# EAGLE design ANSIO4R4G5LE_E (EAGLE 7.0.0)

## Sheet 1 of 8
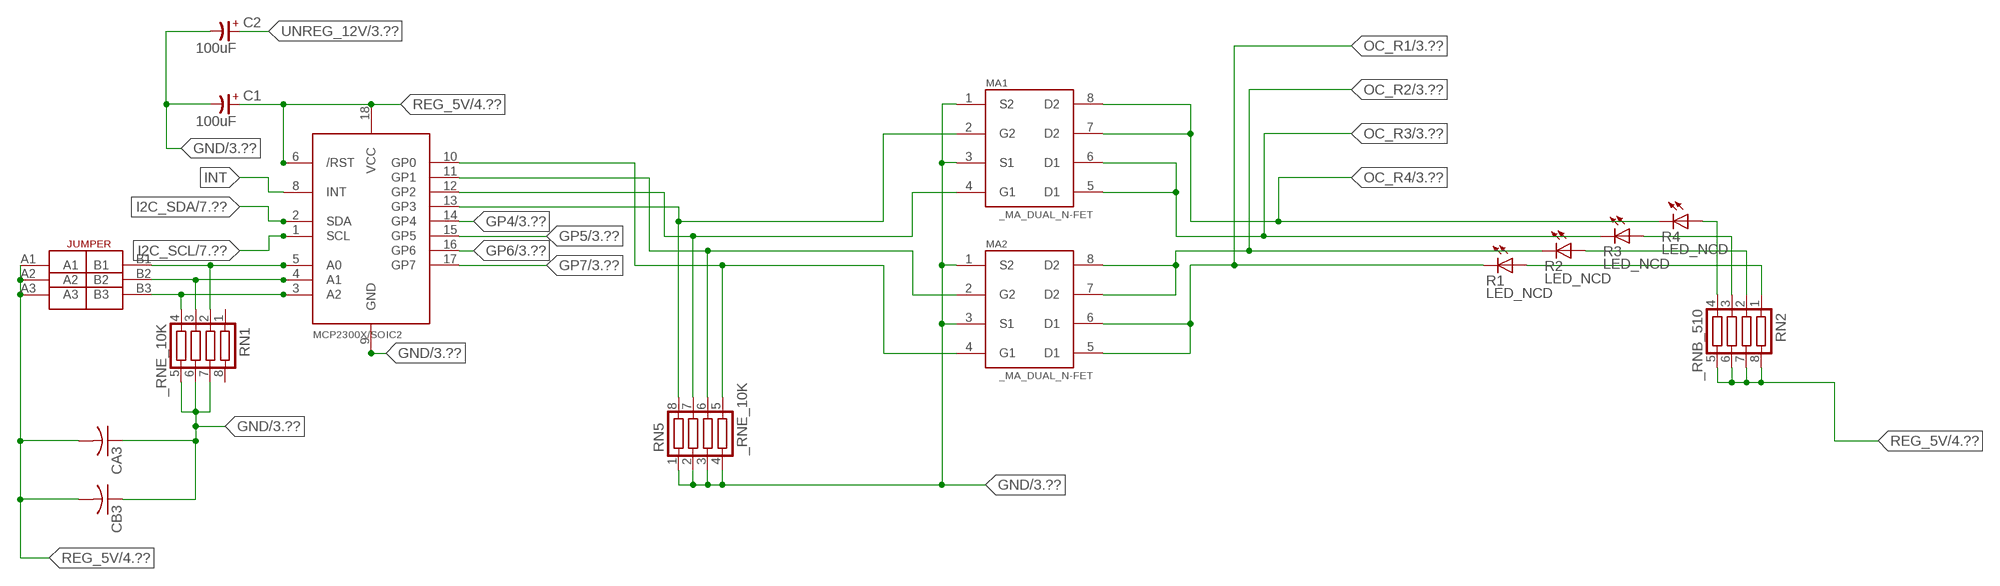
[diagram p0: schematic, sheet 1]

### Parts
C1  100uF  CP-E-025X060  [E-025X060]
C2  100uF  CP-E-025X060  [E-025X060]
CA3  CC1206KRX7R9BB104C1206K  [CC1206KRX7R9BB104]
CB3  TMK316F106ZL-TC1206K  [TMK316F106ZL-T]
IC2  MCP2300X/SO  [SO18W]
MA1  _MA_DUAL_N-FET  [_MA_DUAL_N-FET]
MA2  _MA_DUAL_N-FET  [_MA_DUAL_N-FET]
R1  LED_NCD  [CHIPLED_0603]
R2  LED_NCD  [CHIPLED_0603]
R3  LED_NCD  [CHIPLED_0603]
R4  LED_NCD  [CHIPLED_0603]
RN1  _RNE_10K  [RNE]
RN2  _RNB_510  [RNB]
RN5  _RNE_10K  [RNE]
U$18  JUMPER_3X2  [JUMPER_3X2]

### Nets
GND: C1.- C2.- CA3.1 CB3.1 IC2.9(GND) MA1.1(S2) MA1.3(S1) MA2.1(S2) MA2.3(S1) RN1.5 RN1.6 RN1.7 RN5.1 RN5.2 RN5.3 RN5.4 ; also sheet 3,4,6,7,8
GP4: IC2.14(GP4) ; also sheet 3
GP5: IC2.15(GP5) ; also sheet 3
GP6: IC2.16(GP6) ; also sheet 3
GP7: IC2.17(GP7) ; also sheet 3
I2C_SCL: IC2.1(SCL) ; also sheet 7,8
I2C_SDA: IC2.2(SDA) ; also sheet 4,7,8
INT: IC2.8(INT)
N$6: IC2.5(A0) RN1.2 U$18.B1
N$7: IC2.4(A1) RN1.3 U$18.B2
N$8: IC2.3(A2) RN1.4 U$18.B3
N$20: IC2.13(GP3) MA1.2(G2) RN5.8
N$21: IC2.12(GP2) MA1.4(G1) RN5.7
N$22: IC2.11(GP1) MA2.2(G2) RN5.6
N$23: IC2.10(GP0) MA2.4(G1) RN5.5
N$29: R4.A RN2.4
N$30: R3.A RN2.3
N$31: R2.A RN2.2
N$32: R1.A RN2.1
OC_R1: MA2.5(D1) MA2.6(D1) R1.C ; also sheet 3
OC_R2: MA2.7(D2) MA2.8(D2) R2.C ; also sheet 3
OC_R3: MA1.5(D1) MA1.6(D1) R3.C ; also sheet 3
OC_R4: MA1.7(D2) MA1.8(D2) R4.C ; also sheet 3
REG_5V: C1.+ CA3.2 CB3.2 IC2.6(/RST) IC2.18(VCC) RN2.5 RN2.6 RN2.7 RN2.8 U$18.A1 U$18.A2 U$18.A3 ; also sheet 4,6,7,8
UNREG_12V: C2.+ ; also sheet 3,4
Unconnected: RN1.1 RN1.8

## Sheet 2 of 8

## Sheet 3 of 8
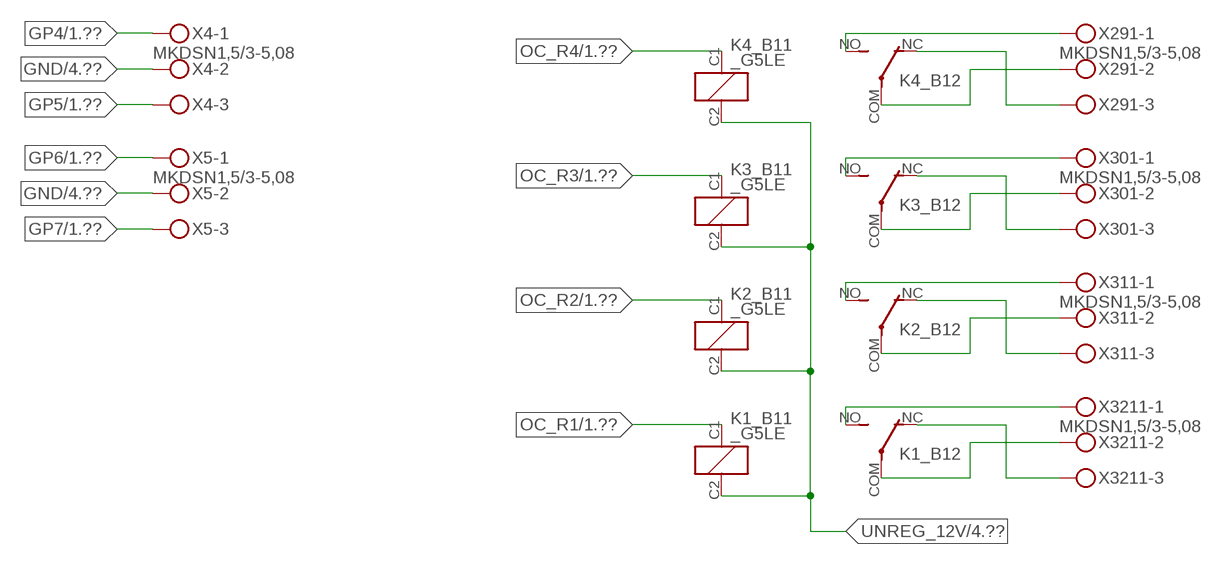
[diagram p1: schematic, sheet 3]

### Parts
K1_B1  _G5LE  [G5LE]
K2_B1  _G5LE  [G5LE]
K3_B1  _G5LE  [G5LE]
K4_B1  _G5LE  [G5LE]
X4  MKDSN1,5/3-5,08  [MKDSN1,5/3-5,08]
X5  MKDSN1,5/3-5,08  [MKDSN1,5/3-5,08]
X291  MKDSN1,5/3-5,08  [MKDSN1,5/3-5,08]
X301  MKDSN1,5/3-5,08  [MKDSN1,5/3-5,08]
X311  MKDSN1,5/3-5,08  [MKDSN1,5/3-5,08]
X3211  MKDSN1,5/3-5,08  [MKDSN1,5/3-5,08]

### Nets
GND: X4.2 X5.2 ; also sheet 1,4,6,7,8
GP4: X4.1 ; also sheet 1
GP5: X4.3 ; also sheet 1
GP6: X5.1 ; also sheet 1
GP7: X5.3 ; also sheet 1
N$215: K4_B1.NO(2:NO) X291.1
N$216: K4_B1.NC(2:NC) X291.3
N$217: K4_B1.COM(2:COM) X291.2
N$218: K3_B1.NO(2:NO) X301.1
N$219: K3_B1.NC(2:NC) X301.3
N$220: K3_B1.COM(2:COM) X301.2
N$221: K2_B1.NO(2:NO) X311.1
N$222: K2_B1.NC(2:NC) X311.3
N$223: K2_B1.COM(2:COM) X311.2
N$224: K1_B1.NO(2:NO) X3211.1
N$225: K1_B1.NC(2:NC) X3211.3
N$226: K1_B1.COM(2:COM) X3211.2
OC_R1: K1_B1.C1(1:C1) ; also sheet 1
OC_R2: K2_B1.C1(1:C1) ; also sheet 1
OC_R3: K3_B1.C1(1:C1) ; also sheet 1
OC_R4: K4_B1.C1(1:C1) ; also sheet 1
UNREG_12V: K1_B1.C2(1:C2) K2_B1.C2(1:C2) K3_B1.C2(1:C2) K4_B1.C2(1:C2) ; also sheet 1,4

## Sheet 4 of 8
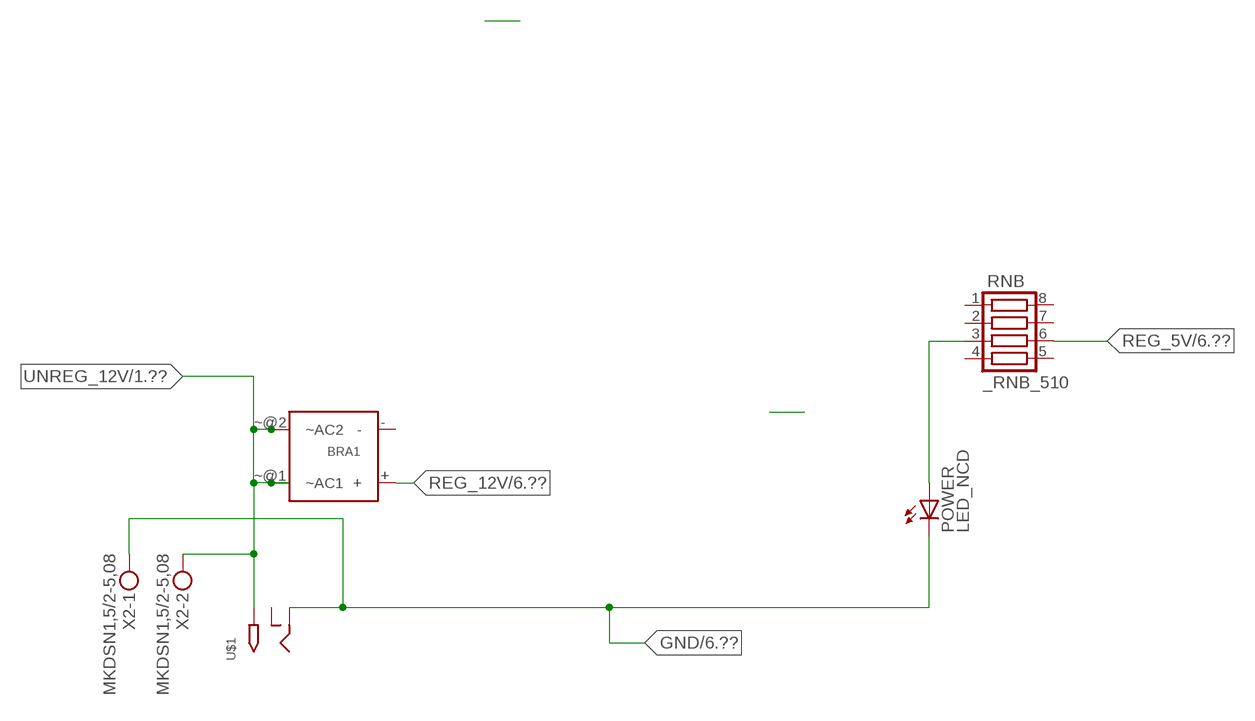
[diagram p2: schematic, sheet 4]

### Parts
BRA1  MB2S_  [MB2S]
POWER  LED_NCD  [CHIPLED_0603]
RNB  _RNB_510  [RNB]
U$1  2.1MMJACK  [PJ-102A]
X2  MKDSN1,5/2-5,08  [MKDSN1,5/2-5,08]

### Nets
GND: POWER.C U$1.RING X2.1 ; also sheet 1,3,6,7,8
N$2: POWER.A RNB.3
REG_5V: RNB.6 ; also sheet 1,6,7,8
REG_12V: BRA1.+ ; also sheet 6
UNREG_12V: BRA1.~@1(~AC1) BRA1.~@2(~AC2) U$1.TIP X2.2 ; also sheet 1,3
Unconnected: BRA1.- RNB.1 RNB.2 RNB.4 RNB.5 RNB.7 RNB.8 U$1.RING_SW

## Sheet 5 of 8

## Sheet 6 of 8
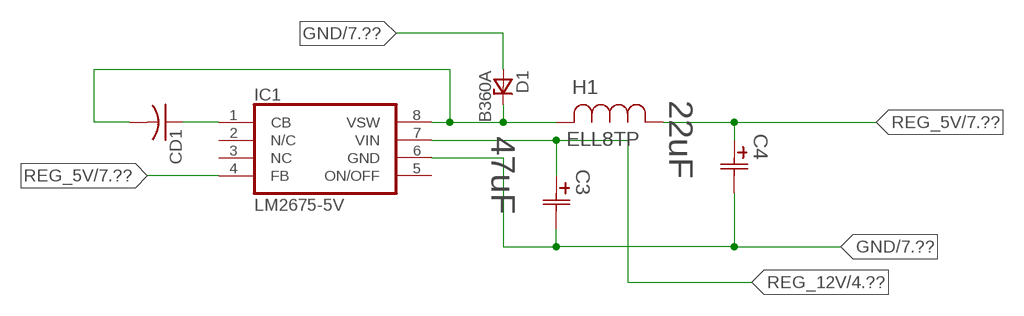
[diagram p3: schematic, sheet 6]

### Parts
C3  47uF  490-5463-6-NDCAP  [C2917(7343)-Y]
C4  22uF  490-5463-6-NDCAP  [C2917(7343)-Y]
CD1  _CD_10NF_50VC1206K  [_CD_10NF_50V]
D1  B360A  [DO214AC_ZENER]
H1  ELL8TP  [IND_ELL8TP]
IC1  LM2675-5V  LM2675  [SO-8]

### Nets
GND: C3.2(C2) C4.2(C2) D1.A IC1.6(GND) ; also sheet 1,3,4,7,8
N$1: CD1.2 D1.C H1.2 IC1.8(VSW)
N$3: CD1.1 IC1.1(CB)
REG_5V: C4.1(C1) H1.1 IC1.4(FB) ; also sheet 1,4,7,8
REG_12V: C3.1(C1) IC1.7(VIN) ; also sheet 4
Unconnected: IC1.2(N/C) IC1.5(ON/OFF)

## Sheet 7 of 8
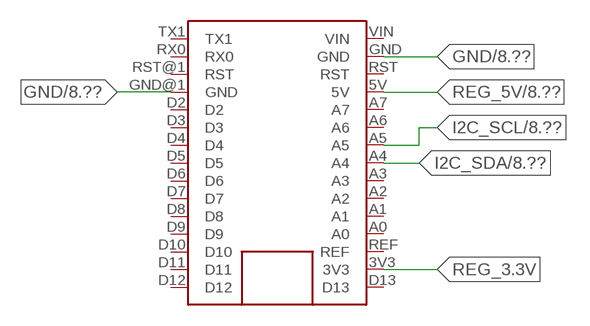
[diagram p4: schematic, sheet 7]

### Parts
FOR_NANO  ARDUINO_NANO  [ARDUINO_NANO]

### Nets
GND: FOR_NANO.GND FOR_NANO.GND@1(GND) ; also sheet 1,3,4,6,8
I2C_SCL: FOR_NANO.A5 ; also sheet 1,8
I2C_SDA: FOR_NANO.A4 ; also sheet 1,4,8
REG_3.3V: FOR_NANO.3V3
REG_5V: FOR_NANO.5V ; also sheet 1,4,6,8
Unconnected: FOR_NANO.A0 FOR_NANO.A1 FOR_NANO.A2 FOR_NANO.A3 FOR_NANO.A6 FOR_NANO.A7 FOR_NANO.D2 FOR_NANO.D3 FOR_NANO.D4 FOR_NANO.D5 FOR_NANO.D6 FOR_NANO.D7 FOR_NANO.D8 FOR_NANO.D9 FOR_NANO.D10 FOR_NANO.D11 FOR_NANO.D12 FOR_NANO.D13 FOR_NANO.REF FOR_NANO.RST FOR_NANO.RST@1(RST) FOR_NANO.RX0 FOR_NANO.TX1 FOR_NANO.VIN

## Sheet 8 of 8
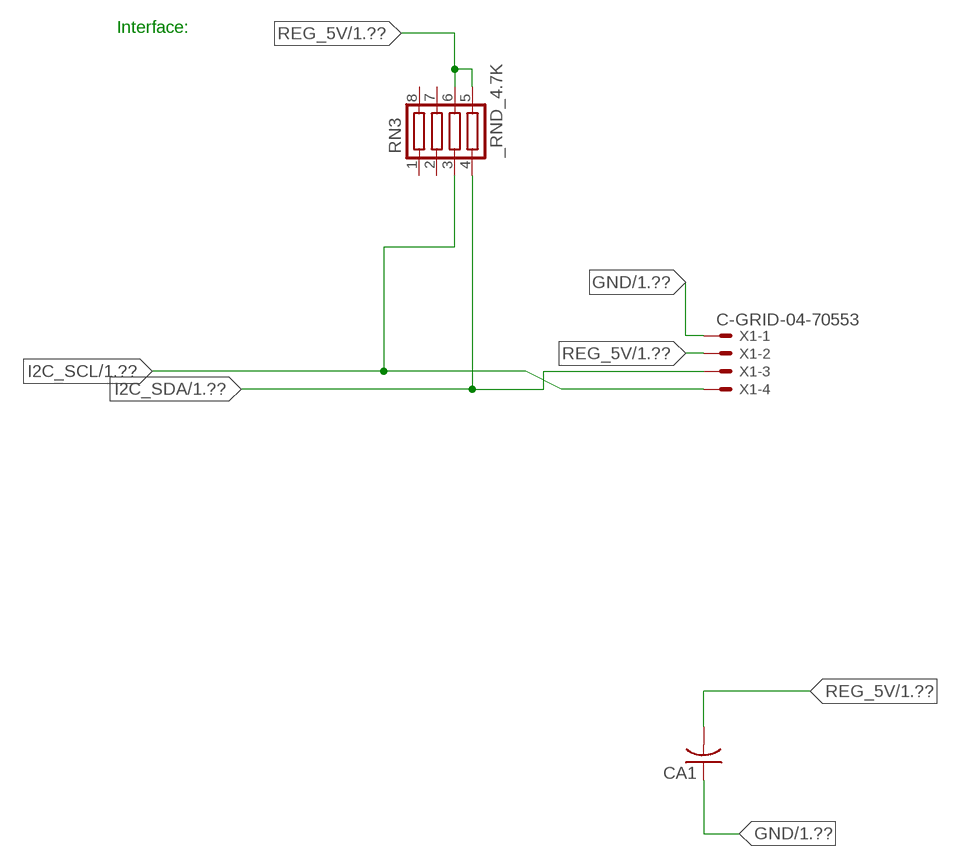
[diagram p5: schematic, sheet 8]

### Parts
CA1  CC1206KRX7R9BB104  [.1UF]
RN3  _RND_4.7K  [RND]
X1  C-GRID-04-70553  [70553-04]

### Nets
GND: CA1.1 X1.1 ; also sheet 1,3,4,6,7
I2C_SCL: RN3.3 X1.4 ; also sheet 1,7
I2C_SDA: RN3.4 X1.3 ; also sheet 1,4,7
REG_5V: CA1.2 RN3.5 RN3.6 X1.2 ; also sheet 1,4,6,7
Unconnected: RN3.1 RN3.2 RN3.7 RN3.8

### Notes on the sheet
- Interface:

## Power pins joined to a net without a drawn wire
NC: IC1.3(NC)

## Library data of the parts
BRA1 = NCD_ULTIMATE_LIBRARY:MB2S: Bridge Rectifier BRA MB2S 200V 500ma Digikey MB2S-TPMSTR-ND/MB2S-TP
C1 C2 = NCD_ULTIMATE_LIBRARY:CP-: Capacitors All Kinds POLARIZED CAP
C3 C4 = NCD_ULTIMATE_bhaskar:490-5463-6-ND: NCD CAP
CA1 CA3 = NCD_ULTIMATE_LIBRARY:CC1206KRX7R9BB104: Capacitor CA .1uF 50V SMT C1206K CC1206KRX7R9BB104
CB3 = NCD_ULTIMATE_LIBRARY:TMK316F106ZL-T: Capacitor CB 10uF SMT 1206 TMK316F106ZL-T
CD1 = NCD_ULTIMATE_LIBRARY:_CD_10NF_50V: Capacitor 10nF SMT
D1 = NCD_ULTIMATE_bhaskar:B360A: NCD DIODE B350A/B360A
FOR_NANO = NCD_ULTIMATE_CONNECTORS:ARDUINO_NANO
H1 = NCD_ULTIMATE_bhaskar:ELL8TP: NCD coil
IC1 = NCD_ULTIMATE_bhaskar:LM2675: LM2675 NCD http://www.ti.com/lit/ds/symlink/lm2675.pdf
IC2 = NCD_ULTIMATE_LIBRARY:MCP2300X: Semiconductor Port Expander I/O 8-Bit I2C MCP23008 Inexpensive i2c i/o expander - 8 general purpose i/o pins with optional pullups
K1_B1 K2_B1 K3_B1 K4_B1 = NCD_ULTIMATE_LIBRARY:_G5LE: Relay 5A/10A SPDT; OC_FARNELL: unknown; OC_NEWARK: unknown
MA1 MA2 = NCD_ULTIMATE_LIBRARY:_MA_DUAL_N-FET: FET Dual N-Channel 8-SOIC NMOSFET Digikey 785-1064-2-ND/AO4842
POWER = NCD_ULTIMATE_bhaskar:LED_NCD
R1-R4 = NCD_ULTIMATE_LIBRARY:LED_NCD: LED Digikey 754-1132-2-ND/APT2012SRCPRV
RN1 RN5 = NCD_ULTIMATE_LIBRARY:_RNE_10K: Resistor Array RNE SMT 10K x 4 Single Resistor Source: http://www.ctscorp.com/components/Datasheets/CTSChipArrayDs.pdf Digikey 742C083103JPTR-ND/742C083103JP; OC_FARNELL: unknown; OC_NEWARK: unknown
RN2 RNB = NCD_ULTIMATE_LIBRARY:_RNB_510: Resistor Array RNB SMT 510 x 4 Single Resistor Source: http://www.ctscorp.com/components/Datasheets/CTSChipArrayDs.pdf Digikey 742C083511JPTR-ND/ 742C083511JP; OC_FARNELL: unknown; OC_NEWARK: unknown
RN3 = NCD_ULTIMATE_LIBRARY:_RND_4.7K: Resistor Array RND SMT 4.7K x 4 Single Resistor Source: http://www.ctscorp.com/components/Datasheets/CTSChipArrayDs.pdf Digikey 742C083472JPTR-ND/742C083472JP; OC_FARNELL: unknown; OC_NEWARK: unknown
U$1 = NCD_ULTIMATE_CONNECTORS:2.1MMJACK: 2.1mm x 5.5mm DC jack with internal switch. Digikey part #PJ-102A, 4UCON part #05537 By microbuilder.eu
U$18 = NCD_ULTIMATE_CONNECTORS:JUMPER_3X2
X1 = NCD_ULTIMATE_CONNECTORS:C-GRID-04: CONNECTOR 4-Pos I2C wire to board 2.54 mm (0.100") pitch header Digikey WM1342-ND/0015912045; OC_FARNELL: unknown; OC_NEWARK: unknown
X2 = NCD_ULTIMATE_CONNECTORS:MKDSN1,5/2-5,08: MKDSN 1,5/ 2-5,08 Printklemme
X4 X5 X291 X301 X311 X3211 = NCD_ULTIMATE_CONNECTORS:MKDSN1,5/3-5,08: MKDSN 1,5/ 3-5,08 Printklemme Nennstrom: 13,5 A Nennspannung: 250 V Rastermaß: 5,08 mm Polzahl: 3 Anschlussart: Schraubanschluss Montage: Löten Anschlussrichtung Leiter/Platine: 0 ° Artikelnummer: 1729131 Source: http://eshop.phoenixcontact.com .. 1729131.pdf

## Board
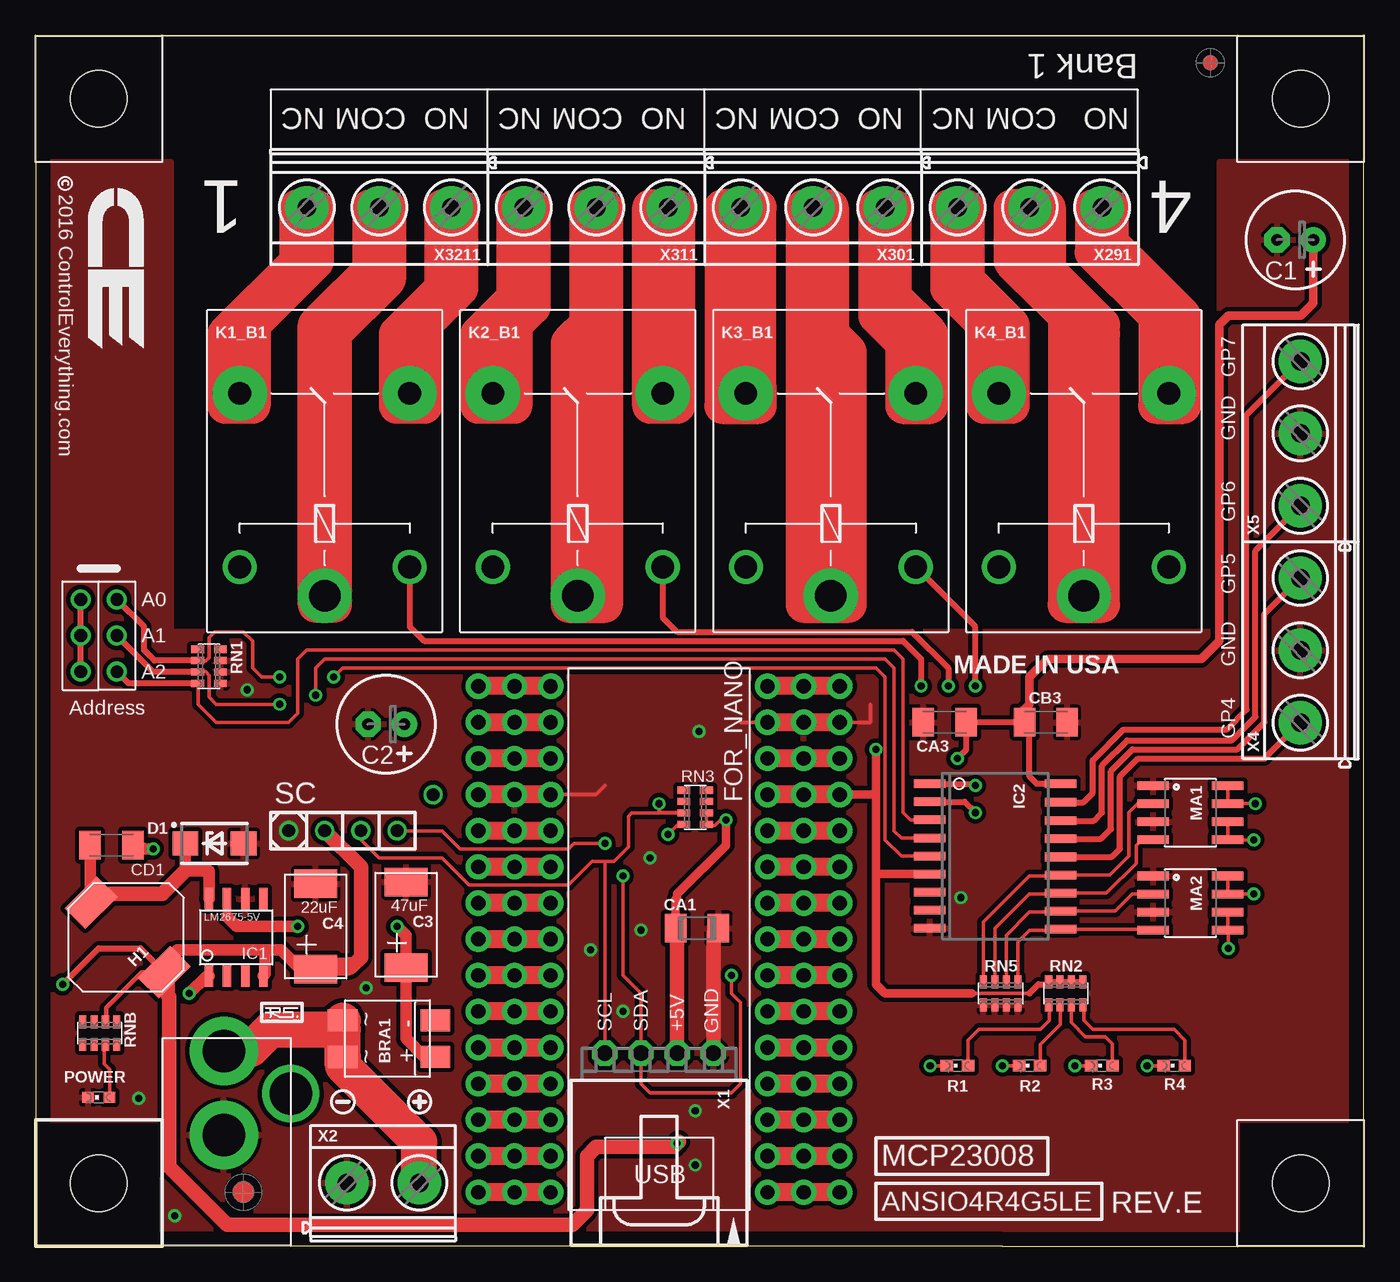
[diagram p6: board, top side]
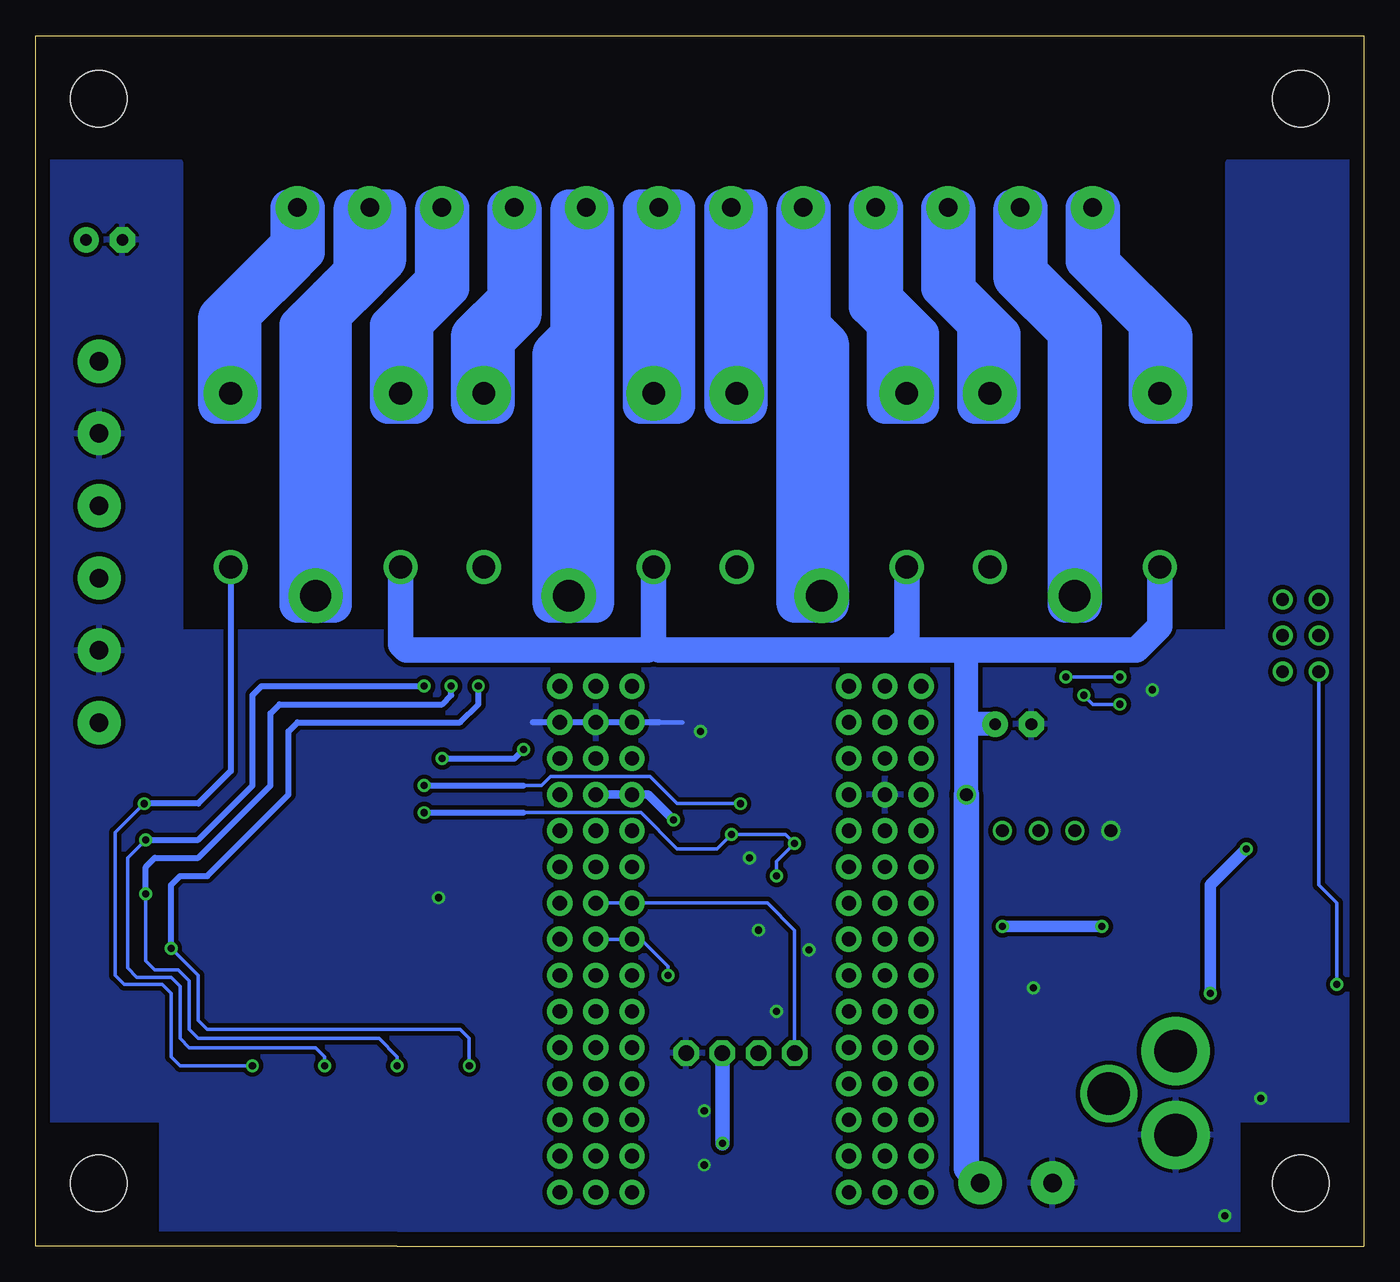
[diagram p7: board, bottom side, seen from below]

Size 93.34 x 85.09 mm. Coordinates in mm from the lower left corner, seen from the top.
Outline: 0,65.71 0,64.77
Outline: 0,64.77 0,0 67.94,0 93.34,0 93.34,85.09 0,85.09 0,64.77
Copper layers (1*16): Top 0.035mm / dielectric 1.5mm / Bottom 0.035mm
Design rules "default": minimum track width 10mil, minimum drill 24mil, track to track 8mil, track to pad 8mil, pad to pad 8mil, via to via 8mil, smd to smd 8mil, copper to edge 40mil, drill to drill 8mil, minimum pad ring 10mil, minimum via ring 8mil, stop-mask expansion 4mil, vias tented up to drill 0mil, thermal gap 10mil
Holes 3.96 mm at 4.45,4.45 4.45,4.45

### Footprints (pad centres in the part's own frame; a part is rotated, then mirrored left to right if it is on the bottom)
MB2S = smd 1.55 x 2.1: + 0,-6.5; - 2.54,-6.5; ~@1 0,0; ~@2 2.54,0
E-025X060 = drill 0.813 pad 1.778: + -1.27,0 | drill 0.813 pad 1.778 octagon: - 1.27,0
C2917(7343)-Y = smd 2 x 3: 1 -3,0; 2 3,0
.1UF = smd 1.5 x 2: 1 -1.5,0; 2 1.5,0
CC1206KRX7R9BB104 = smd 1.5 x 2: 1 -1.5,0; 2 1.5,0
TMK316F106ZL-T = smd 1.5 x 2: 1 -1.5,0; 2 1.5,0
_CD_10NF_50V = smd 1.5 x 2: 1 -1.5,0; 2 1.5,0
DO214AC_ZENER = smd 1.8 x 1.7: A 2.05,0; C -2.05,0
ARDUINO_NANO = drill 1 pad 1.778: 3V1 -2.54,-2.54; 3V3 0,-2.54; 5V 0,-27.94; 5V1 -2.54,-27.94; A0 0,-7.62; A1 0,-10.16; A2 0,-12.7; A3 0,-15.24; A4 0,-17.78; A5 0,-20.32; A6 0,-22.86; A7 0,-25.4; A8 -2.54,-7.62; A9 -2.54,-10.16; A10 -2.54,-12.7; A11 -2.54,-15.24; A12 -2.54,-17.78; A13 -2.54,-20.32; A14 -2.54,-22.86; A15 -2.54,-25.4; D1 -2.54,0; D2 20.32,-25.4; D3 20.32,-22.86; D4 20.32,-20.32; D5 20.32,-17.78; D6 20.32,-15.24; D7 20.32,-12.7; D8 20.32,-10.16; D9 20.32,-7.62; D10 20.32,-5.08; D11 20.32,-2.54; D12 20.32,0; D13 0,0; D14 22.86,0; D15 22.86,-2.54; D16 22.86,-5.08; D17 22.86,-7.62; D18 22.86,-10.16; D19 22.86,-12.7; D20 22.86,-15.24; D21 22.86,-17.78; D22 22.86,-20.32; D23 22.86,-22.86; D24 22.86,-25.4; GND 0,-33.02; GND1 -2.54,-33.02; GND@1 20.32,-27.94; GND@2 22.86,-27.94; P$16 2.54,0; P$17 2.54,-2.54; P$18 2.54,-5.08; P$19 2.54,-7.62; P$20 2.54,-10.16; P$21 2.54,-12.7; P$22 2.54,-15.24; P$23 2.54,-17.78; P$24 2.54,-20.32; P$25 2.54,-22.86; P$26 2.54,-25.4; P$27 2.54,-27.94; P$28 2.54,-30.48; P$29 2.54,-33.02; P$30 2.54,-35.56; P$31 17.78,0; P$32 17.78,-2.54; P$33 17.78,-5.08; P$34 17.78,-7.62; P$35 17.78,-10.16; P$36 17.78,-12.7; P$37 17.78,-15.24; P$38 17.78,-17.78; P$39 17.78,-20.32; P$40 17.78,-22.86; P$41 17.78,-25.4; P$42 17.78,-27.94; P$43 17.78,-30.48; P$44 17.78,-33.02; P$45 17.78,-35.56; REF 0,-5.08; REF1 -2.54,-5.08; RST 0,-30.48; RST1 -2.54,-30.48; RST@1 20.32,-30.48; RST@2 22.86,-30.48; RX0 20.32,-33.02; RX1 22.86,-33.02; TX1 20.32,-35.56; TX2 22.86,-35.56; VIN 0,-35.56; VIN1 -2.54,-35.56
IND_ELL8TP = smd 2.054 x 3.2 rotated 45: 1 -2.442,-2.696; 2 2.442,2.442
SO-8 = smd 0.6 x 1.55: 1 -1.905,-2.69; 2 -0.635,-2.69; 3 0.635,-2.69; 4 1.905,-2.69; 5 1.905,2.71; 6 0.635,2.71; 7 -0.635,2.71; 8 -1.905,2.71
SO18W = smd 0.6 x 2.2: 1 -4.445,-4.6; 2 -3.175,-4.6; 3 -1.905,-4.6; 4 -0.635,-4.6; 5 0.635,-4.6; 6 1.905,-4.6; 7 3.175,-4.6; 8 4.445,-4.6; 9 5.715,-4.6; 10 5.775,4.6; 11 4.505,4.6; 12 3.235,4.6; 13 1.965,4.6; 14 0.695,4.6; 15 -0.575,4.6; 16 -1.845,4.6; 17 -3.145,4.6; 18 -4.445,4.6
G5LE = drill 1.6: C1 -7.493,-5.969; C2 -7.493,5.969 | drill 2.2 pad 3.81: COM -9.525,0 | drill 1.6 pad 3.81: NC 4.699,5.969; NO 4.699,-5.969
_MA_DUAL_N-FET = smd 0.61 x 2.21: 1 -1.905,-2.616; 2 -0.635,-2.616; 3 0.635,-2.616; 4 1.905,-2.616; 5 1.905,2.616; 6 0.635,2.616; 7 -0.635,2.616; 8 -1.905,2.616
CHIPLED_0603 = smd 0.8 x 0.8: A 0,-0.75; C 0,0.75
CHIPLED_0603' = smd 0.8 x 0.876: A 0,-0.75; C 0,0.75
RNE = smd 0.5 x 0.9: 1 -1.2,-0.8; 2 -0.4,-0.8; 3 0.4,-0.8; 4 1.2,-0.8; 5 1.2,0.8; 6 0.4,0.8; 7 -0.4,0.8; 8 -1.2,0.8
RNB = smd 0.5 x 0.9: 1 -1.2,-0.8; 2 -0.4,-0.8; 3 0.4,-0.8; 4 1.2,-0.8; 5 1.2,0.8; 6 0.4,0.8; 7 -0.4,0.8; 8 -1.2,0.8
RND = smd 0.5 x 0.9: 1 -1.2,-0.8; 2 -0.4,-0.8; 3 0.4,-0.8; 4 1.2,-0.8; 5 1.2,0.8; 6 0.4,0.8; 7 -0.4,0.8; 8 -1.2,0.8
PJ-102A = drill 3 pad 4.8: RING 0.1,-3.39; TIP 0.1,-9.29 | drill 3 pad 3.251: RING_SW -4.6,-6.29
PCB_MOUNTING_HOLE = hole 3.962: 4.445,4.445
JUMPER_3X2 = drill 0.9: A1 0,5.08; A2 0,2.54; A3 0,0; B1 2.54,5.08; B2 2.54,2.54; B3 2.54,0
70553-04 = drill 1.1 pad 1.778 octagon: 1 -3.81,-7.62; 2 -1.27,-7.62; 3 1.27,-7.62; 4 3.81,-7.62
MKDSN1,5/2-5,08 = drill 1.3 pad 3.048: 1 -2.561,0.025; 2 2.519,0.025
MKDSN1,5/3-5,08 = drill 1.3 pad 3.048: 1 -7.641,0.025; 2 -2.561,0.025; 3 2.519,0.025

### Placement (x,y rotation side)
BRA1  21.59,13.34 90 top
C1  88.52,70.74 180 top
C2  24.64,36.7 180 top
C3  26.04,22.61 90 top
C4  19.68,22.48 90 top
CA1  46.48,22.35 180 top
CA3  63.88,36.83 0 top
CB3  70.99,36.83 180 top
CD1  5.33,28.19 180 top
D1  12.57,28.32 0 top
FOR_NANO  53.98,3.81 180 top
H1  6.35,21.72 90 top
IC1  14.1,21.72 0 top
IC2  67.44,28.07 270 top
K1_B1  20.32,55.24 90 top
K2_B1  38.1,55.24 90 top
K3_B1  55.88,55.24 90 top
K4_B1  73.66,55.24 90 top
MA1  81.15,30.48 270 top
MA2  81.15,24.13 270 top
POWER  4.45,10.48 90 top
R1  LED_NCD  [CHIPLED_0603']  64.77,12.7 90 top
R2  LED_NCD  [CHIPLED_0603']  69.85,12.7 90 top
R3  LED_NCD  [CHIPLED_0603']  74.93,12.7 90 top
R4  LED_NCD  [CHIPLED_0603']  80.01,12.7 90 top
RN1  12.19,40.77 270 top
RN2  72.39,17.78 0 top
RN3  46.35,30.86 270 top
RN5  67.82,17.78 0 top
RNB  4.51,14.99 0 top
U$1  13.34,4.45 180 top
U$2  [VISION_REF15]  14.61,3.81 0 top
U$3  [ICON_MINUS]  21.59,10.16 180 top
U$4  PCB_MOUNTING_HOLE  [PCB_MOUNTING_HOLE]  93.34,76.2 90 top
U$5  [ICON_PLUS]  26.99,10.16 90 top
U$6  PCB_MOUNTING_HOLE  [PCB_MOUNTING_HOLE]  93.34,0 90 top
U$11  PCB_MOUNTING_HOLE  [PCB_MOUNTING_HOLE]  8.89,76.2 90 top
U$18  3.17,40.39 0 top
U$19  [VISION_REF10]  82.55,83.19 0 top
U$21  [ICON_USA]  64.52,40.26 0 top
X1  43.81,5.97 180 top
X2  24.45,4.45 0 top
X4  88.9,44.45 90 top
X5  88.9,59.69 90 top
X291  67.31,73.03 180 top
X301  52.07,73.03 180 top
X311  36.83,73.03 180 top
X3211  21.59,73.03 180 top

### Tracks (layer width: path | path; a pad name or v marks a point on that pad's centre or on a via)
GND  (via drill 0.5, 0.9)
  Top 0.254: 36.2,31.75 39.37,31.75 40.01,32.39 | FOR_NANO.GND@1 32.38,31.75 | 49.53,36.83 56.52,36.83 58.67,36.83 58.67,38.1
  Top 1.016: X1.1 47.62,22
  Bottom 0.254: 51.44,36.83 FOR_NANO.GND
  Bottom 0.305: 47.88,36.83 49.53,36.83 51.44,36.83
  Bottom 0.406: 49.53,36.83 58.42,36.83
  other vias: 14.86,39.12 65.02,24.51 9.78,2.16 17.78,29.21 41.27,16.51 46.35,9.53 46.61,36.2 46.35,5.72 42.55,22.23 38.99,20.83 7.24,10.41 43.18,27.3 23.24,18.16
  pour Bottom (isolate 0.305): -1.91,8.89 8.89,8.89 8.89,0 84.45,0 84.45,8.89 92.71,8.89 92.71,76.2 83.19,76.2 83.19,43.18 9.53,43.18 9.53,76.2 -1.91,76.2
  pour Top (isolate 0.305): -3.17,8.89 8.89,8.89 8.89,0 84.45,0 84.45,8.89 92.71,8.89 92.71,76.2 83.19,76.2 83.19,43.18 9.53,43.18 9.53,76.2 -3.17,76.2
GP4
  Top 0.406: IC2.14 75.63,27.37 76.2,27.94 76.2,33.02 77.47,34.29 86.36,34.29 X4.1
GP5
  Top 0.406: IC2.15 74.87,28.64 75.56,29.34 75.56,33.4 77.09,34.92 84.45,34.92 86.36,36.83 86.36,44.45 X4.3
GP6
  Top 0.406: IC2.16 74.36,29.91 74.93,30.48 74.93,33.78 76.71,35.56 84.07,35.56 85.72,37.21 85.72,48.9 X5.1
GP7
  Top 0.406: IC2.17 73.63,31.21 74.3,31.88 74.3,34.16 76.45,36.32 83.69,36.32 85.09,37.72 85.09,58.42 X5.3
I2C_SCL  (via drill 0.5, 0.9)
  Top 0.254: 40.01,27.05 40.64,27.05 41.66,28.07 41.66,30.23 41.89,30.46 RN3.3 45.54,30.48 43.81,30.48 v43.81,31.12 | 40.01,27.05 39.12,27.05 37.47,25.4 30.48,25.4 28.57,27.3 24.13,27.3 22.86,28.57 v22.86,29.21 | X1.4 40.01,27.05
  Top 0.406: IC2.1 65.91,32.51 v66.04,32.39
  Bottom 0.254: 59.05,32.39 57.78,32.39 57.15,33.02 50.16,33.02 48.26,31.12 v43.81,31.12 | FOR_NANO.A5 41.91,24.13 40.01,22.23 X1.4
  Bottom 0.406: v66.04,32.39 59.05,32.39
I2C_SDA  (via drill 0.5, 0.9)
  Top 0.254: RN3.4 45.16,29.66 v44.45,28.96 | 40,28.33 v40.01,28.32 37.85,28.32 37.47,27.94 29.84,27.94 28.57,29.21 v25.4,29.21 | v41.27,26.04 41.27,19.05 42.55,17.78 X1.3 42.55,11.43 43.18,10.79 48.9,10.79 49.53,11.43 49.53,17.15 48.9,17.78 v48.9,19.05
  Top 0.406: IC2.2 65.28,31.24 v66.04,30.48
  Bottom 0.254: v41.27,26.04 41.27,27.05 v40.01,28.32 40.64,28.96 v44.45,28.96 45.47,27.94 48.26,27.94 50.8,30.48 59.05,30.48 | v48.9,19.05 48.9,19.69 50.8,21.59 FOR_NANO.A4
  Bottom 0.406: v66.04,30.48 59.05,30.48
N$1
  Top 0.813: H1.2 3.88,24.77 | D1.C 10.52,26.4 12.19,26.38 IC1.8 | CD1.2 3.83,24.15 4.45,24.77
  Top 1.016: 3.88,24.77 4.45,24.77 8.89,24.77 10.52,26.4
N$2
  Top 0.254: POWER.A 5.2,12.46 4.83,12.83 4.83,14.1 RNB.3
  Top 0.406: 4.95,14.14 RNB.3
N$3  (via drill 0.5)
  Top 0.813: IC1.1 12.04,19.03 v10.79,17.78 | v8.26,27.94 7.72,27.94 CD1.1
  Bottom 0.813: v10.79,17.78 10.79,25.4 v8.26,27.94
N$6  (via drill 0.5)
  Top 0.254: IC2.5 60.83,27.43 59.69,28.57 59.69,40 59.05,40.64 21.59,40.64 v20.95,40 | v17.14,40 15.88,40 15.24,40.64 15.24,42.55 14.61,43.18 12.57,43.18 12.19,42.8 12.19,41.4 11.94,41.15 11.41,41.15 RN1.2
  Top 0.406: RN1.2 8.36,41.17 7.62,41.91 7.62,43.56 U$18.B1
  Bottom 0.254: v20.95,40 v17.14,40
N$7  (via drill 0.5)
  Top 0.254: IC2.4 60.83,28.7 60.33,29.21 60.33,40.64 59.69,41.27 20.32,41.27 19.68,40.64 v19.68,38.73 | v17.14,38.1 12.7,38.1 12.19,38.61 12.19,40.13 11.94,40.39 11.41,40.39 RN1.3
  Top 0.406: RN1.3 8.27,40.37 U$18.B2
  Bottom 0.254: v19.68,38.73 19.05,38.1 v17.14,38.1
N$8
  Top 0.254: IC2.3 61.47,29.97 60.96,30.48 60.96,41.27 60.33,41.91 19.05,41.91 18.41,41.27 18.41,37.47 17.78,36.83 12.7,36.83 11.43,38.1 11.43,39.53 RN1.4
  Top 0.406: RN1.4 6.53,39.57 U$18.B3
N$20
  Top 0.254: MA1.2 77.47,31.12 76.83,30.48 76.83,27.43 75.5,26.1 IC2.13 71.97,26.04 69.85,26.04 66.62,22.8 RN5.8
N$21
  Top 0.254: MA1.4 77.72,28.57 77.34,28.19 77.34,26.92 75.25,24.83 IC2.12 71.97,24.77 69.85,24.77 67.42,22.33 RN5.7
N$22
  Top 0.254: MA2.2 77.09,24.77 75.89,23.56 IC2.11 71.97,23.5 69.85,23.5 68.22,21.86 RN5.6
N$23
  Top 0.254: MA2.4 78.6,22.29 IC2.10 71.97,22.23 69.85,22.23 69.02,21.39 RN5.5
N$29
  Top 0.254: R4.A 80.76,14.49 80.01,15.24 74.3,15.24 73.66,15.88 73.66,16.91 RN2.4
N$30
  Top 0.254: R3.A 75.68,14.24 75.18,14.73 73.79,14.73 72.77,15.75 72.77,16.96 RN2.3
N$31
  Top 0.254: R2.A 70.6,14.21 72.01,15.62 72.01,16.96 RN2.2
N$32
  Top 0.254: R1.A 65.52,14.47 66.29,15.24 70.61,15.24 71.25,15.88 71.25,16.92 RN2.1
N$215
  Top 2.54: X291.1 74.95,69.83 79.38,65.41 79.38,60.2 K4_B1.NO
N$216
  Top 2.54: X291.3 64.79,67.29 67.31,64.77 67.31,60.33 K4_B1.NC
N$217
  Top 2.54: X291.2 69.87,68.56 73.66,64.77 K4_B1.COM
N$218
  Top 2.54: X301.1 59.71,65.38 61.59,63.5 61.59,60.2 K3_B1.NO
N$219
  Top 2.54: X301.3 49.55,60.94 50.16,60.33 50.16,60.2 K3_B1.NC
N$220
  Top 2.54: X301.2 54.63,46.97 K3_B1.COM
N$221
  Top 2.54: X311.1 44.47,60.35 K2_B1.NO
N$222
  Top 2.54: X311.3 34.31,66.06 32.38,64.13 32.38,60.2 K2_B1.NC
N$223
  Top 2.54: X311.2 39.39,47.01 K2_B1.COM
N$224
  Top 2.54: X3211.1 29.23,67.33 26.04,64.13 26.04,60.2 K1_B1.NO
N$225
  Top 2.54: X3211.3 19.07,69.24 13.97,64.13 13.97,60.33 K1_B1.NC
N$226
  Top 2.54: X3211.2 24.15,68.6 20.32,64.77 K1_B1.COM
N$316
  Top 2.54: 74.95,73 74.95,69.83 79.38,65.41 79.38,60.2 79.63,59.94
N$317
  Top 2.54: 64.79,73 64.79,67.92 67.31,65.41 67.31,60.33 67.69,59.94
N$318
  Top 2.54: 69.87,73 69.87,69.19 73.66,65.41 73.66,45.72
N$319
  Top 2.54: 59.71,73 59.71,65.38 61.59,63.5 61.59,60.2 61.85,59.94
N$320
  Top 2.54: 49.55,73 49.55,60.3 49.91,59.94
N$321
  Top 2.54: 54.63,73 54.63,46.97 55.88,45.72
N$322
  Top 2.54: 44.47,73 44.47,60.35 44.07,59.94
N$323
  Top 2.54: 34.31,73 34.31,66.06 32.38,64.13 32.38,60.2 32.13,59.94
N$324
  Top 2.54: 39.39,73 39.39,47.01 38.1,45.72
N$325
  Top 2.54: 29.23,73 29.23,67.33 26.67,64.77 26.67,60.33 26.29,59.94
N$326
  Top 2.54: 19.07,73 19.07,69.24 14.61,64.77 14.61,60.2 14.35,59.94
N$327
  Top 2.54: 24.15,73 24.15,68.6 20.32,64.77 20.32,45.72
N$328
  Bottom 2.54: 20.32,45.72 20.32,64.13 24.13,67.94 24.13,72.98 24.15,73
N$329
  Bottom 2.54: 14.35,59.94 14.35,64.52 19.05,69.22 19.05,72.98 19.07,73
N$330
  Bottom 2.54: 26.29,59.94 26.29,63.75 29.21,66.67 29.21,72.98 29.23,73
N$331
  Bottom 2.54: 44.07,59.94 44.07,62.48 44.45,62.87 44.45,72.98 44.47,73
N$332
  Bottom 2.54: 61.85,59.94 61.85,63.25 59.69,65.41 59.69,72.98 59.71,73
N$333
  Bottom 2.54: 32.13,59.94 32.13,63.25 34.29,65.41 34.29,72.98 34.31,73
N$334
  Bottom 2.54: 38.1,45.72 38.1,64.13 39.37,65.41 39.37,72.98 39.39,73
N$335
  Bottom 2.54: 49.91,59.94 49.91,62.48 49.53,62.87 49.53,71.71 49.55,73
N$336
  Top 2.54: 49.53,62.23 49.53,73.03 50.16,73.03 50.16,62.23 | 49.53,62.23 50.16,62.23 | 50.16,62.23 50.16,61.59 | 50.16,61.59 50.16,59.69 49.53,59.69 49.53,60.33 | 49.53,60.33 49.53,61.59 | 49.53,62.23 49.53,61.59 | 49.53,61.59 50.16,61.59 | 49.53,60.33 50.8,60.33 | 50.8,60.33 50.8,73.03 48.26,73.03 48.26,59.05 50.8,59.05 50.8,60.33
N$337
  Top 2.54: 54.61,73.03 54.61,64.13 | 55.88,62.87 55.88,45.72 | 54.61,73.03 55.88,73.03 55.88,64.13 | 55.88,64.13 55.88,62.87 | 55.88,62.87 54.61,64.13 | 54.61,64.13 54.61,45.09 | 54.61,45.09 57.15,45.09 57.15,62.87 55.88,64.13 | 54.61,73.03 53.98,73.03 53.98,45.09 54.61,45.09
N$338
  Top 2.54: 59.05,66.04 59.05,73.03 60.33,73.03 60.33,66.67 62.87,64.13 62.87,59.05 60.96,59.05 60.96,63.5 | 59.05,66.04 60.96,64.13 60.96,63.5 | 59.05,66.04 59.05,65.41 60.96,63.5
N$339
  Top 2.54: 66.67,59.05 66.67,64.77 64.14,67.31 64.14,73.03 65.41,73.03 65.41,67.94 68.58,64.77 68.58,59.05 66.67,59.05
N$340
  Top 2.54: 69.85,73.03 68.58,73.03 68.58,69.22 71.12,66.67 | 71.12,66.67 72.39,65.41 72.39,45.09 74.93,45.09 74.93,64.13 | 74.93,64.13 69.85,69.22 69.85,73.03 | 69.85,73.03 71.12,73.03 71.12,68.58 | 71.12,68.58 71.12,66.67 | 74.93,64.13 74.93,64.77 71.12,68.58
N$341
  Top 2.54: 74.3,73.03 74.3,69.85 78.74,65.41 78.74,59.05 80.64,59.05 80.64,65.41 75.56,70.48 75.56,73.03 74.3,73.03
N$342
  Top 2.54: 45.09,73.03 45.09,59.05 43.18,59.05 43.18,73.03 45.09,73.03
N$343
  Top 2.54: 40.01,73.03 40.01,45.09 37.47,45.09 37.47,63.5 38.73,64.77 38.73,73.03 40.01,73.03
N$344
  Top 2.54: 34.92,73.03 34.92,66.04 33.66,64.77 33.66,59.05 31.11,59.05 31.11,64.13 33.66,66.67 33.66,73.03 34.92,73.03
N$345
  Top 2.54: 29.21,73.03 29.84,73.03 29.84,67.31 27.3,64.77 27.3,59.05 25.4,59.05 25.4,64.13 28.57,67.31 | 29.21,67.94 29.21,73.03 | 29.21,73.03 28.57,73.03 28.57,66.67
N$346
  Top 2.54: 24.77,68.58 24.77,73.03 24.13,73.03 | 24.77,68.58 23.5,67.31 | 23.5,67.31 20.95,64.77 20.95,64.13 | 20.95,64.13 20.95,45.09 19.68,45.09 19.68,64.77 24.13,69.22 24.13,73.03 | 24.13,73.03 23.5,73.03 23.5,67.31 | 24.77,68.58 24.77,67.94 20.95,64.13
N$347
  Top 2.54: 19.68,73.03 19.68,69.22 15.24,64.77 15.24,59.05 13.34,59.05 13.34,64.13 18.41,69.22 18.41,73.03 19.68,73.03
N$348
  Bottom 2.54: 19.05,73.03 18.41,73.03 18.41,69.22 13.34,64.13 13.34,59.05 15.24,59.05 15.24,64.77 19.68,69.22 19.68,73.03
N$349
  Bottom 2.54: 23.5,73.03 23.5,68.58 19.68,64.77 19.68,45.09 20.95,45.09 20.95,64.13 24.77,67.94 24.77,73.03 23.5,73.03
N$350
  Bottom 2.54: 28.57,73.03 28.57,67.31 25.4,64.13 25.4,59.05 27.3,59.05 27.3,64.77 29.84,67.31 29.84,73.03 28.57,73.03
N$351
  Bottom 2.54: 33.66,73.03 33.66,66.67 31.11,64.13 31.11,59.05 33.66,59.05 33.66,64.77 34.92,66.04 34.92,73.03 33.66,73.03
N$352
  Bottom 2.54: 38.73,73.03 38.73,64.77 37.47,63.5 37.47,45.09 40.01,45.09 40.01,73.03 38.73,73.03
N$353
  Bottom 2.54: 45.09,73.03 43.18,73.03 43.18,59.05 45.09,59.05 45.09,73.03
N$354
  Bottom 2.54: 48.26,73.03 48.26,59.05 50.8,59.05 50.8,73.03 48.26,73.03
N$355
  Bottom 2.54: 53.98,73.03 53.98,45.09 57.15,45.09 57.15,62.87 55.88,64.13 55.88,73.03 53.98,73.03
N$356
  Bottom 2.54: 59.05,73.03 59.05,65.41 60.96,63.5 60.96,59.05 62.87,59.05 62.87,64.13 60.33,66.67 60.33,73.03 59.05,73.03
N$357
  Bottom 2.54: 67.69,59.94 67.69,63.75 66.67,64.77 | 66.67,64.77 64.77,66.67 | 64.77,66.67 64.77,72.98 64.79,73 | 64.77,66.67 64.14,67.31 64.14,73.03 65.41,73.03 65.41,67.94 68.58,64.77 68.58,59.05 66.67,59.05 66.67,64.77
N$358
  Bottom 2.54: 73.66,45.72 73.66,64.13 72.39,65.41 | 72.39,65.41 69.85,67.94 | 69.85,67.94 69.85,72.98 69.87,73 | 69.85,67.94 68.58,69.22 68.58,73.03 71.12,73.03 71.12,68.58 74.93,64.77 74.93,45.09 72.39,45.09 72.39,65.41
N$359
  Bottom 2.54: 79.63,59.94 79.63,64.52 78.74,65.41 | 78.74,65.41 74.93,69.22 | 74.93,69.22 74.93,72.98 74.95,73 | 74.93,69.22 74.3,69.85 74.3,73.03 75.56,73.03 75.56,70.48 80.64,65.41 80.64,59.05 78.74,59.05 78.74,65.41
N$521
  Bottom 2.54: 54.61,72.98 54.63,73
N$522
  Bottom 2.54: 55.88,45.72 55.88,62.87 54.61,64.13
OC_R1  (via drill 0.5)
  Top 0.254: R1.C v62.87,12.7 | v83.82,20.95 83.82,22.15 MA2.5 MA2.6
  Top 0.406: K1_B1.C1 26.29,43.56 27.3,42.55 60.96,42.55 62.23,41.27 v62.23,39.37
  Bottom 0.254: v62.87,12.7 62.87,14.61 63.5,15.24 81.28,15.24 81.92,15.88 81.92,19.05 v83.82,20.95
  Bottom 0.406: v83.82,20.95 83.82,25.4 83.19,26.04 81.28,26.04 75.56,31.75 75.56,36.2 74.93,36.83 63.5,36.83 62.23,38.1 v62.23,39.37
OC_R2  (via drill 0.5)
  Top 0.254: R2.C v67.94,12.7 | v85.6,24.77 MA2.7 MA2.8
  Top 0.406: K2_B1.C1 44.07,44.2 45.09,43.18 61.59,43.18 64.14,40.64 v64.14,39.37
  Bottom 0.254: v67.94,12.7 67.94,13.34 69.22,14.61 81.92,14.61 82.55,15.24 82.55,18.67 83.31,19.43 84.96,19.43 85.6,20.07 v85.6,24.77
  Bottom 0.406: v85.6,24.77 85.6,26.67 84.96,27.3 81.92,27.3 76.83,32.39 76.83,37.47 76.2,38.1 64.77,38.1 64.14,38.73 v64.14,39.37
OC_R3  (via drill 0.5)
  Top 0.254: R3.C v73.03,12.7 | v85.6,28.57 MA1.5 MA1.6
  Top 0.406: v66.04,39.37 66.04,43.56 K3_B1.C1
  Bottom 0.254: v73.03,12.7 73.03,13.34 73.66,13.97 82.55,13.97 83.19,14.61 83.19,18.29 83.82,18.92 86.23,18.92 86.87,19.56 86.87,27.3 v85.6,28.57
  Bottom 0.406: v85.6,28.57 81.92,28.57 78.11,32.39 78.11,38.73 77.47,39.37 v66.04,39.37
OC_R4  (via drill 0.5)
  Top 0.254: R4.C v78.11,12.7 | v85.72,31.12 MA1.7 MA1.8
  Bottom 0.254: v78.11,12.7 83.19,12.7 83.82,13.34 83.82,17.78 84.45,18.41 87.12,18.41 87.76,19.05 87.76,29.08 v85.72,31.12
  Bottom 0.406: K4_B1.C1 79.63,33.4 81.92,31.12 v85.72,31.12
REG_5V  (via drill 0.5, 0.9)
  Top 0.229: 65.79,17.78 69.85,17.78
  Top 0.254: RN3.6 RN3.5 47.23,29.59 47.75,29.59 48.13,29.97 v48.51,29.97 | 44.98,24.41 45.09,24.51
  Top 0.305: H1.1 7.46,19.27 4.95,16.76 4.95,15.83 RNB.6
  Top 0.406: U$18.A3 U$18.A2 U$18.A1 | IC2.18 70.36,32.51 69.85,33.02 69.85,36.47 CB3.2 CA3.2 65.38,34.9 v64.77,34.29 | 69.85,17.78 70.48,18.41 71.03,18.41 RN2.8 RN2.7 RN2.6 RN2.5 | v1.91,18.41 4.45,20.95 7.37,20.95 H1.1
  Top 0.61: v59.05,34.92 59.05,31.75 | C1.+ 89.79,66.29 88.9,65.41 83.82,65.41 83.19,64.77 83.19,42.55 81.92,41.27 71.12,41.27 69.85,40 69.85,38.1 69.22,37.47 69.22,37.11 CB3.2 | 59.05,26.04 59.05,18.41 59.69,17.78 65.79,17.78 | 59.05,26.04 59.05,31.75 | FOR_NANO.5V 59.05,31.75 | CA1.2 44.98,24.41 | 45.09,24.51 45.09,24.77 48.51,28.19 v48.51,29.97 | IC2.6 59.18,26.16 59.05,26.04
  Top 0.813: 16.13,20.83 9.96,20.83 H1.1 | 16.13,20.83 17.27,20.83 18.41,19.69 20.75,19.69 C4.1 | IC1.4 16.13,19.15 16.13,20.83
  Top 1.016: H1.1 9.27,18.41 9.27,17.65 9.4,17.53 9.4,5.59 13.46,1.52 37.72,1.52 38.73,2.54 38.73,6.35 39.37,6.99 44.83,6.99 v45.09,7.24 45.21,7.37 | 22.05,19.69 22.23,19.69 22.86,20.32 22.86,26.67 v20.32,29.21 | X1.2 45.09,22.25 CA1.2
  Top 1.27: 20.75,19.69 22.05,19.69
  Bottom 0.254: v1.91,18.41 1.91,24.13 3.17,25.4 U$18.A3
  Bottom 0.406: v64.77,34.29 59.69,34.29 v59.05,34.92
  Bottom 0.61: FOR_NANO.5V 50.29,31.75 v48.51,29.97
  Bottom 1.016: v45.09,7.24 X1.2
REG_12V  (via drill 0.5)
  Top 0.61: IC1.7 13.46,23.16 | 14.1,22.48 14.15,22.48
  Top 0.813: v18.41,22.48 14.15,22.48 13.46,23.16 | v25.4,22.48 26.04,21.84 C3.1 26.04,14.61 27.3,13.34 BRA1.+
  Bottom 0.813: v18.41,22.48 v25.4,22.48
UNREG_12V  (via drill 0.9)
  Top 2.54: X2.2 26.97,7.32 21.59,12.7 BRA1.~@1 21.59,15.24 | 21.59,15.24 BRA1.~@2 | U$1.TIP 15.14,13.87 16.51,15.24 21.59,15.24
  Bottom 1.676: v27.94,31.75 27.94,36.83 | 27.94,36.83 27.94,41.91 | C2.+ 27.81,36.7 27.94,36.83
  Bottom 1.778: 33.02,41.91 49.53,41.91 49.91,42.29 | 33.02,41.91 27.94,41.91 16,41.91 14.35,43.56 K1_B1.C2 | K2_B1.C2 32.13,42.8 33.02,41.91 | K3_B1.C2 49.91,42.29 | K4_B1.C2 67.69,42.29 67.31,41.91 50.29,41.91 49.91,42.29 | v27.94,31.75 27.94,5.44 X2.2

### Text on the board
tNames: Bank 1 | NC | COM | NO | NC | COM | NO | NC | COM | NO | NC | COM | NO | 1 | 4 | 2016 ControlEverything.com | GP7 | GND | GP6 | GP5 | A0 | A1 | GND | A2 | Address | GP4 | SC | SCL | SDA | +5V | GND | MCP23008 | ANSIO4R4G5LE | REV.E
